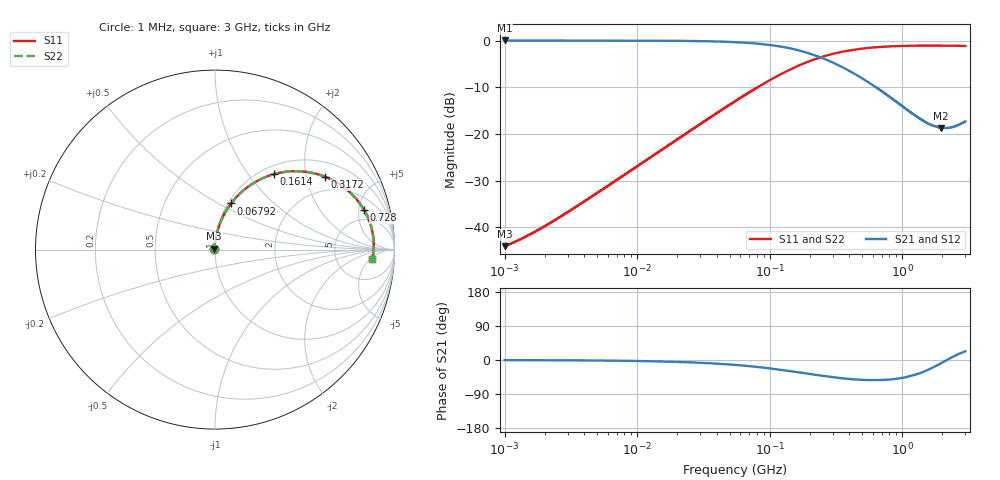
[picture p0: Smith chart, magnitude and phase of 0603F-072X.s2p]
!s-Parameter Generated by FASTRON Sdn. Bhd.
!FASTRON P/N : 0603F-072X
!Keysight Technologies: E4991B_MY54100416_A.01.15
!Date: Thu Jun 20 13:04:32 2024
!Version  :Rev00  Thu Jun 20 13:04:32 2024
!Data & Calibration Information:
!Freq  S11  S21  S12  S22
!PortZ  Port1:50+j0  Port2:50+j0
!When reading reference impedance value at option line is always used.
! Remarks : This data is being provided solely for informational purposes.
# Hz S dB R 50
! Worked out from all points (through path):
!   1601 points, 1 MHz to 3 GHz, reference 50 ohm
!   highest |S21| = 0.03 dB at 1 MHz (marker M1); lowest = -18.7 dB at 1.961 GHz (marker M2)
!   group delay of S21, straight-line fit = 8.01 ps
!   lowest |S11| = -44.0 dB at 1 MHz (marker M3), VSWR 1.01, Z = 49.6 + j0.493 ohm
!   |S11| at or under -10 dB: start of sweep to 80.92 MHz
!   |S22| runs from -44.0 to -1.1 dB; largest |S21 - S12| = 0
!   S11 on the Smith chart (normalised r, x): 1 MHz: 0.99, +0.01; 67.92 MHz: 1.03, +0.57; 161.4 MHz: 1.14, +1.33; 317.2 MHz: 1.46, +2.58; 728 MHz: 3.40, +5.73; 3 GHz: 12, -6
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1000000  -44.00 128.0  0.03 -0.3  0.03 -0.3  -44.00 128.0
1641145  -41.10 114.0  0.03 -0.5  0.03 -0.5  -41.10 114.0
3804036  -34.80 98.7  0.03 -1.0  0.03 -1.0  -34.80 98.7
1.447069e7  -23.90 86.3  -0.02 -3.7  -0.02 -3.7  -23.90 86.3
2.944989e7  -18.00 80.9  -0.11 -7.2  -0.11 -7.2  -18.00 80.9
5.504702e7  -13.00 73.9  -0.33 -13.0  -0.33 -13.0  -13.00 73.9
6.792166e7  -11.30 70.8  -0.48 -15.7  -0.48 -15.7  -11.30 70.8
1.044488e8  -8.19 62.7  -1.00 -22.8  -1.00 -22.8  -8.19 62.7
1.288778e8  -6.82 57.9  -1.41 -27.0  -1.41 -27.0  -6.82 57.9
1.614254e8  -5.49 52.1  -2.01 -31.9  -2.01 -31.9  -5.49 52.1
2.083556e8  -4.21 45.2  -2.92 -37.7  -2.92 -37.7  -4.21 45.2
2.583764e8  -3.33 39.1  -3.90 -42.4  -3.90 -42.4  -3.33 39.1
3.172153e8  -2.67 33.5  -5.02 -46.4  -5.02 -46.4  -2.67 33.5
4.75755e8  -1.79 23.4  -7.73 -52.0  -7.73 -52.0  -1.79 23.4
7.279565e8  -1.31 14.8  -11.20 -52.5  -11.20 -52.5  -1.31 14.8
7.925923e8  -1.25 13.3  -11.90 -51.7  -11.90 -51.7  -1.25 13.3
1.070143e9  -1.12 8.6  -14.60 -45.3  -14.60 -45.3  -1.12 8.6
1.444887e9  -1.07 4.7  -17.20 -31.4  -17.20 -31.4  -1.07 4.7
1.637435e9  -1.06 3.1  -18.00 -22.7  -18.00 -22.7  -1.06 3.1
1.960646e9  -1.06 1.1  -18.70 -8.8  -18.70 -8.8  -1.06 1.1
2.324278e9  -1.08 -0.7  -18.60 5.5  -18.60 5.5  -1.08 -0.7
3e9  -1.15 -3.5  -17.30 23.0  -17.30 23.0  -1.15 -3.5
